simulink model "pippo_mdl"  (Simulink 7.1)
settings: Solver=ode45  StartTime=0.0  StopTime=10.0  RelTol=1e-3
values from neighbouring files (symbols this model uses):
  bm = 0.02*N*m*sec/rad    (= 0.02)    [pippo.m]
  Cr = 0*N*m    (= 0)    [pippo.m]
  Ia_0 = 0*A    (= 0)    [pippo.m]
  Ia_max = 10000000*A    (= 10000000)    [pippo.m]
  Jm = 0.5*Kg*m^2    (= 0.5)    [pippo.m]
  Km = 1    [pippo.m]
  La = 10*mHenry    (= 0.01)    [pippo.m]
  Ra = 2*Ohm    (= 2)    [pippo.m]
  Tc = Tfin/2000    (= 5e-05)    [pippo.m]
  Va = 100*V    (= 100)    [pippo.m]
  Wm_0 = 0*rpm    (= 0)    [pippo.m]

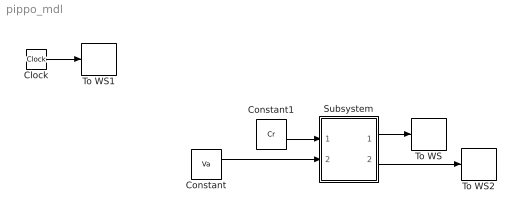
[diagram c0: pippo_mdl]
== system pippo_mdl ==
  Clock : Clock
  Constant : Constant  Value=Va  OutDataType=sfix(16)  OutScaling=2^0
  Constant1 : Constant  Value=Cr  OutDataType=sfix(16)  OutScaling=2^0
  Subsystem : Subsystem
  To WS : ToWorkspace  VariableName=Ia  SampleTime=Tc  SaveFormat=Array
  To WS1 : ToWorkspace  VariableName=t  SampleTime=Tc  SaveFormat=Array
  To WS2 : ToWorkspace  VariableName=Wm  SampleTime=Tc  SaveFormat=Array
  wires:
  Constant/1 -> Subsystem/2(Va)
  Clock/1 -> To WS1/1
  Constant1/1 -> Subsystem/1(Tr)
  Subsystem/1(Ia) -> To WS/1
  Subsystem/2(Wm) -> To WS2/1

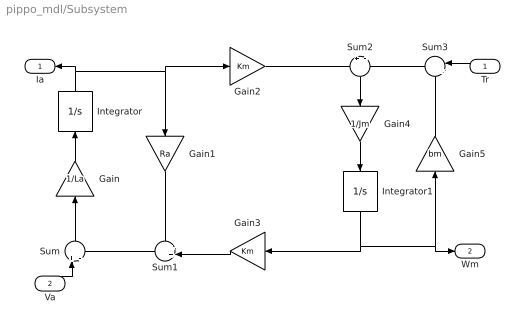
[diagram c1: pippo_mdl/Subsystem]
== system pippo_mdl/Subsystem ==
  Tr : Inport  Orientation=left
  Va : Inport  Orientation=up  Port=2
  Gain : Gain  Orientation=up  Gain=1/La  ParameterDataType=sfix(16)  ParameterScaling=2^0  OutDataType=sfix(16)  OutScaling=2^0
  Gain1 : Gain  Orientation=down  Gain=Ra  ParameterDataType=sfix(16)  ParameterScaling=2^0  OutDataType=sfix(16)  OutScaling=2^0
  Gain2 : Gain  Gain=Km  ParameterDataType=sfix(16)  ParameterScaling=2^0  OutDataType=sfix(16)  OutScaling=2^0
  Gain3 : Gain  Orientation=left  Gain=Km  ParameterDataType=sfix(16)  ParameterScaling=2^0  OutDataType=sfix(16)  OutScaling=2^0
  Gain4 : Gain  Orientation=down  Gain=1/Jm  ParameterDataType=sfix(16)  ParameterScaling=2^0  OutDataType=sfix(16)  OutScaling=2^0
  Gain5 : Gain  Orientation=up  Gain=bm  ParameterDataType=sfix(16)  ParameterScaling=2^0  OutDataType=sfix(16)  OutScaling=2^0
  Integrator : Integrator  Orientation=up  InitialCondition=Ia_0  LimitOutput=on  UpperSaturationLimit=Ia_max  LowerSaturationLimit=-Ia_max
  Integrator1 : Integrator  Orientation=down  InitialCondition=Wm_0
  Sum : Sum  Orientation=up  Inputs=+|-  OutDataType=sfix(16)  OutScaling=2^0
  Sum1 : Sum  Orientation=left  Inputs=++|  OutDataType=sfix(16)  OutScaling=2^0
  Sum2 : Sum  Orientation=down  Inputs=+|-  OutDataType=sfix(16)  OutScaling=2^0
  Sum3 : Sum  Orientation=left  Inputs=|++  OutDataType=sfix(16)  OutScaling=2^0
  Ia : Outport  Orientation=left
  Wm : Outport  Port=2
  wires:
  Sum/1 -> Gain/1
  Gain/1 -> Integrator/1
  Integrator/1 -> Gain1/1, Gain2/1, Ia/1
  Sum1/1 -> Sum/2
  Gain1/1 -> Sum1/1
  Gain3/1 -> Sum1/2
  Gain2/1 -> Sum2/1
  Sum2/1 -> Gain4/1
  Gain4/1 -> Integrator1/1
  Integrator1/1 -> Gain3/1, Gain5/1, Wm/1
  Gain5/1 -> Sum3/2
  Sum3/1 -> Sum2/2
  Tr/1 -> Sum3/1
  Va/1 -> Sum/1
